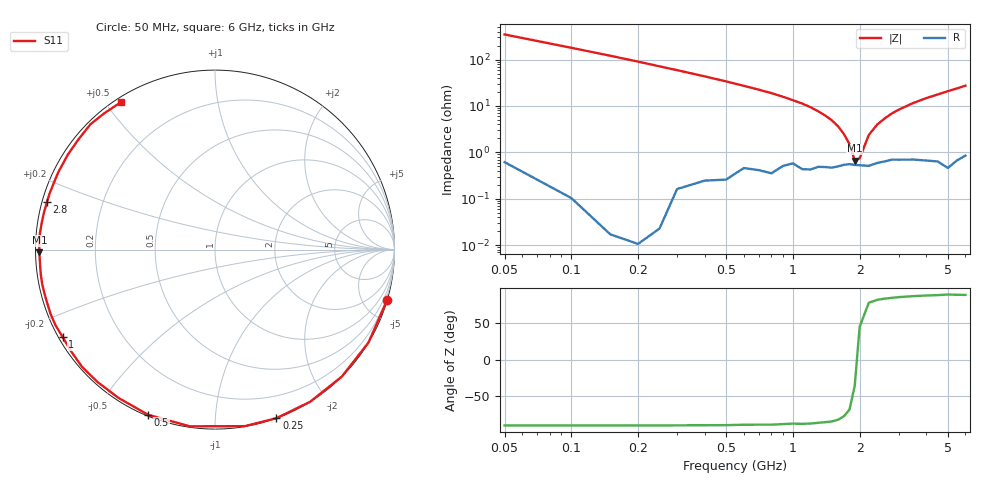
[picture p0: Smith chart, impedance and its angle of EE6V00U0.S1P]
! Infineon Technologies  Discrete & RF Semiconductors
! BBY55-02W
! Si Tuning Diode in SCD-80
! VR = 6 V
! S-Parameters:  June  2000
# GHz  S  MA  R  50
!  f  S11
! GHz  MAG  ANG
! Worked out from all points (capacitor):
!   34 points, 50 MHz to 6 GHz, reference 50 ohm
!   read as one part to ground: C = 8.86 pF near 50 MHz
!   lowest |Z| = 664 mohm at 1.9 GHz (marker M1)
!   series resonance near 1.943 GHz, so ESL is about 760 pH
!   S11 on the Smith chart (normalised r, x): 50 MHz: 0.01, -6.94; 250 MHz: 0.00, -1.43; 500 MHz: 0.01, -0.67; 1 GHz: 0.01, -0.27; 2.8 GHz: 0.01, +0.14; 6 GHz: 0.02, +0.55
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0.05  0.9995 -16.4
0.1  0.9997 -31.2
0.15  0.9999 -45.0
0.2  0.9999 -58.0
0.25  0.9997 -70.0
0.3  0.9973 -80.5
0.4  0.9944 -98.1
0.5  0.9929 -112.0
0.6  0.9859 -123.0
0.7  0.9863 -131.6
0.8  0.9877 -138.6
0.9  0.9817 -144.9
1  0.9785 -150.2
1.1  0.9836 -154.6
1.2  0.9836 -158.7
1.3  0.9811 -162.6
1.6  0.9803 -171.8
1.7  0.9787 -174.5
1.9  0.9788 -179.1
2.2  0.9798 174.7
2.4  0.9768 171.0
2.8  0.973 164.3
3.5  0.9738 153.8
4  0.9758 147.1
4.5  0.9776 141.1
5  0.9844 134.8
5.5  0.9784 129.0
6  0.9742 122.6
